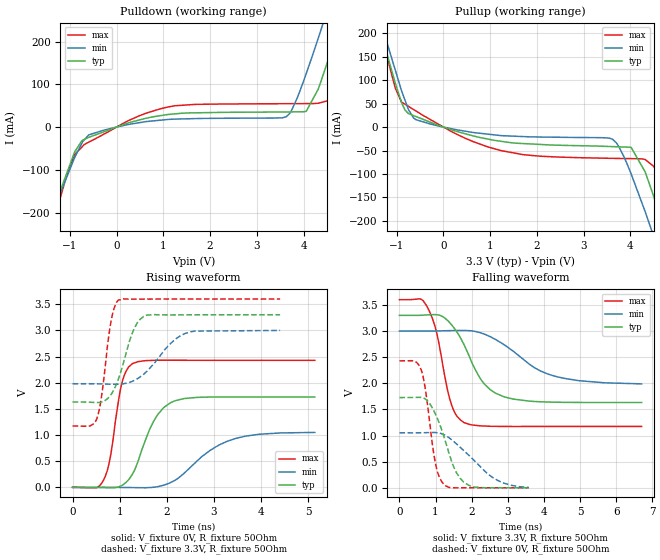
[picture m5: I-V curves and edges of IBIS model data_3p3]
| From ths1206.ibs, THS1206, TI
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|   data_3p3 Model
[Model]   data_3p3
Model_type   Output
Polarity   Non-Inverting
Vmeas = 1.65
Vref = 1.65
Cref = 2pF
Rref = 50
|   typ   min   max
|   (nom PVT)   (fast PVT)   (slow PVT)
C_comp   1.924e-12   1.914e-12   2.001e-12
|ON state : BUFFER OUTPUT TURNED HIGH
|C_comp   1.924e-12   1.914e-12   2.001e-12
|OFF state: BUFFER OUTPUT TURNED LOW
|C_comp   1.784e-12   1.775e-12   1.813e-12
| Where nom  PVT is Nominal Process, 3.3V, 43C
|   Fast PVT is Strong Process,  3.6V, -55C
|   Slow PVT is Weak Process,   3V, 145C
[Voltage Range]   3.3   3   3.6
|Ambient Temperature   25   125   -55
|Junction Temperature
[Temperature Range]   43   145   -55
[Pullup Reference]   3.3   3   3.6
[Pulldown Reference]   0   0   0
[Power Clamp Reference]   3.3   3   3.6
[GND Clamp Reference]   0   0   0
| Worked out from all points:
|   slope of the pulldown table from 0 to 0.495 V, typ, clamps not added: 29.4 ohm
|   slope of the pullup table from 0 to 0.495 V, typ, clamps not added: 32.9 ohm
|   falling waveform, V_fixture 3.3V, R_fixture 50Ohm: 20-80 % time 777ps typ, 1.3ns min, 439ps max; typ from 3.3 V to 1.63 V
|   rising waveform, V_fixture 0V, R_fixture 50Ohm: 20-80 % time 478ps typ, 894ps min, 253ps max; typ from 0 V to 1.73 V
|   rising waveform, V_fixture 3.3V, R_fixture 50Ohm: 20-80 % time 348ps typ, 602ps min, 204ps max; typ from 1.63 V to 3.3 V
|   falling waveform, V_fixture 0V, R_fixture 50Ohm: 20-80 % time 524ps typ, 968ps min, 288ps max; typ from 1.73 V to 0 V
[Pulldown]
|   Voltage   I(typ)   I(min)   I(max)
-3.3V     -914.2mA   -844.7mA   -1.036A
-1.7V     -318.2mA   -306.2mA   -365.5mA
-1.375V   -207.2mA   -206.6mA   -231.9mA
-896.4mV  -58.22mA   -71.31mA   -64.48mA
-591mV    -23.88mA   -18.1mA    -34.96mA
1.098V    29.4mA     17.82mA    46.91mA
3.63V     35.23mA    24.11mA    54.69mA
4.059V    36.98mA    125.2mA    54.89mA
4.468V    137.5mA    259.3mA    60.08mA
4.662V    206mA      325.5mA    95.82mA
5.062V    349.3mA    466.7mA    239.3mA
6.6V      932.6mA    1.03A      847.3mA
[Pullup]
|   Voltage   I(typ)   I(min)   I(max)
-3.3V     971.4mA    955.5mA    1.007A
-1.69V    336.2mA    351.8mA    341.6mA
-1.325V   200.2mA    221.8mA    194.4mA
-896.4mV  52.46mA    77.5mA     53.32mA
-591mV    22.55mA    15.87mA    34.47mA
1.246V    -30.53mA   -18.32mA   -50.45mA
3.618V    -41.67mA   -25.99mA   -66.71mA
4.016V    -43.25mA   -99.85mA   -67.3mA
4.468V    -138.8mA   -224.2mA   -81.29mA
4.691V    -209.3mA   -293mA     -134.2mA
4.877V    -269.2mA   -351.3mA   -203.2mA
6.6V      -898.3mA   -925.7mA   -902.6mA
[Ramp]
R_load = 50
|   typ   min   max
dV/dt_r   1.03604/4.77138e-10   0.631179/8.8993e-10   1.4574/2.51992e-10
dV/dt_f   1.0013/7.7156e-10   0.611526/1.31342e-09   1.45583/4.37549e-10
[Falling Waveform]
V_fixture = 3.3V
V_fixture_min = 3V
V_fixture_max = 3.6V
R_fixture = 50Ohm
|   Time   V(typ)   V(min)   V(max)
0s        3.3V       3V         3.6V
578ps     3.301V     3V         3.613V
764ps     3.308V     3V         3.471V
1.028ns   3.312V     3.001V     2.979V
1.448ns   3.115V     3.008V     1.579V
1.776ns   2.757V     3.01V      1.253V
2.344ns   1.992V     2.943V     1.182V
2.878ns   1.746V     2.747V     1.174V
4.366ns   1.637V     2.124V     1.174V
6.708ns   1.631V     1.988V     1.174V
[Rising Waveform]
V_fixture = 0V
V_fixture_min = 0V
V_fixture_max = 0V
R_fixture = 50Ohm
|   Time   V(typ)   V(min)   V(max)
0s        1.497nV    4.504nV    1.191nV
502ps     -617.5uV   172.4uV    -8.712mV
664ps     -4.323mV   245.3uV    149.2mV
808ps     -8.551mV   41.47uV    607.8mV
1.042ns   34.86mV    -1.505mV   1.973V
1.28ns    266.8mV    -4.365mV   2.368V
1.74ns    1.292V     3.738mV    2.429V
2.178ns   1.655V     136.6mV    2.43V
3.452ns   1.728V     931.7mV    2.429V
5.144ns   1.727V     1.05V      2.429V
[Rising Waveform]
V_fixture = 3.3V
V_fixture_min = 3V
V_fixture_max = 3.6V
R_fixture = 50Ohm
|   Time   V(typ)   V(min)   V(max)
0s        1.631V     1.981V     1.174V
514ps     1.622V     1.979V     1.31V
614ps     1.632V     1.977V     1.731V
822ps     1.78V      1.971V     3.2V
978ps     2.082V     1.972V     3.582V
1.276ns   2.965V     2.029V     3.598V
1.51ns    3.268V     2.163V     3.599V
2.08ns    3.296V     2.749V     3.6V
2.494ns   3.299V     2.971V     3.6V
4.408ns   3.3V       2.999V     3.6V
[Falling Waveform]
V_fixture = 0V
V_fixture_min = 0V
V_fixture_max = 0V
R_fixture = 50Ohm
|   Time   V(typ)   V(min)   V(max)
0s        1.727V     1.052V     2.429V
422ps     1.729V     1.052V     2.422V
604ps     1.729V     1.053V     2.253V
718ps     1.699V     1.055V     1.888V
1ns       1.405V     1.057V     460.7mV
1.204ns   1.038V     1.025V     86.9mV
1.516ns   379.4mV    879.1mV    -38.25uV
1.78ns    109.4mV    713.6mV    421.4uV
2.73ns    1.619mV    137.6mV    109.8uV
3.584ns   361.9uV    6.266mV    124.3uV
